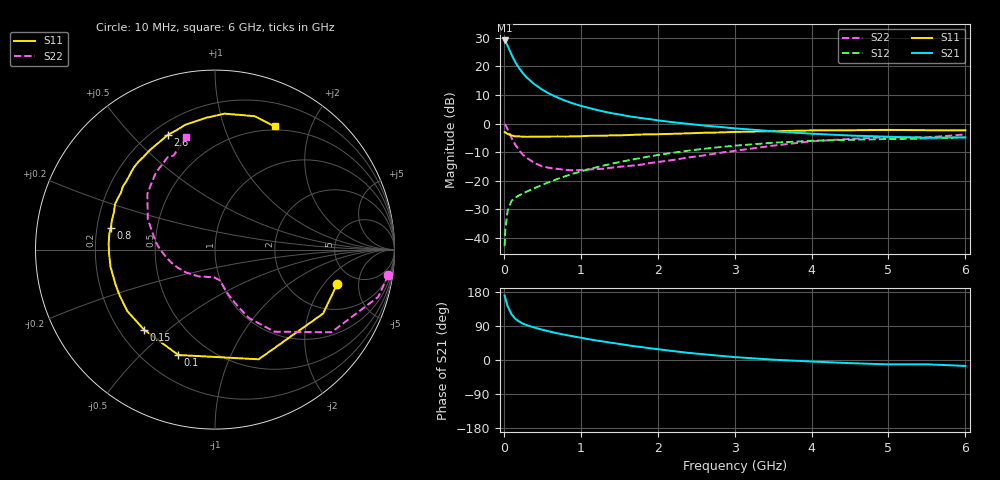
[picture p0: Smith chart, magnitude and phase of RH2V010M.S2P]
! SIEMENS Small Signal Semiconductors
! BFR106
! Si NPN RF Bipolar Junction Transistor in SOT23
! VCE = 2 V  IC = 10 mA
! Common Emitter S-Parameters:  August  1996
# GHz  S  MA  R  50
!  f  S11  S21  S12  S22
! GHz  MAG  ANG  MAG  ANG  MAG  ANG  MAG  ANG
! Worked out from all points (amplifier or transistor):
!   36 points, 10 MHz to 6 GHz, reference 50 ohm
!   highest |S21| = 29.1 dB at 10 MHz (marker M1)
!   |S21| within 3 dB of that: start of sweep to 68.03 MHz
!   unconditionally stable (mu >= 1): 470.6 MHz to 2.33 GHz; 4.596 GHz to end of sweep
!   at 250 MHz: K = 0.72, MSG = 20.9 dB, |S12| = -24.4 dB
!   at 1.4 GHz: K = 1.11, MAG = 6.9 dB, |S12| = -14.0 dB
!   at 6 GHz: K = 1.02, MAG = -0.9 dB, |S12| = -4.8 dB
!   S11 on the Smith chart (normalised r, x): 10 MHz: 3.65, -2.76; 100 MHz: 0.34, -0.65; 150 MHz: 0.30, -0.42; 800 MHz: 0.26, +0.10; 2.6 GHz: 0.26, +0.64; 6 GHz: 0.46, +1.50
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0.01  0.7076 -15.5  28.37 170.4  0.0072 84.3  0.9765 -8.2
0.02  0.6998 -30.6  27.42 162.6  0.0144 77.0  0.9476 -16.1
0.05  0.6577 -68.3  22.78 141.4  0.0304 61.2  0.7955 -35.4
0.1  0.6219 -109.2  16.06 120.6  0.0447 48.5  0.5645 -54.1
0.15  0.596 -131.6  11.76 108.5  0.051 43.6  0.4248 -63.7
0.2  0.5967 -144.8  9.259 101.3  0.0558 44.0  0.3404 -68.1
0.25  0.5898 -153.9  7.513 95.7  0.0606 44.6  0.2825 -71.8
0.3  0.5875 -160.7  6.333 91.8  0.0649 46.6  0.2502 -74.3
0.4  0.5901 -170.6  4.842 85.4  0.0747 50.3  0.2037 -77.8
0.5  0.5905 -177.7  3.903 79.9  0.0849 52.8  0.1787 -80.5
0.6  0.5934 176.7  3.287 74.9  0.0964 55.0  0.1676 -83.4
0.7  0.5954 171.5  2.846 70.3  0.108 56.5  0.1612 -87.5
0.8  0.5936 168.1  2.506 66.3  0.1205 57.3  0.1553 -91.3
1.1  0.6117 155.6  1.883 55.1  0.1583 58.5  0.1578 -104.0
1.3  0.6126 149.1  1.621 48.5  0.1852 57.9  0.1627 -112.8
1.6  0.629 139.7  1.359 39.3  0.2257 55.8  0.1809 -126.8
2.2  0.663 123.1  1.055 23.6  0.3092 48.8  0.231 -154.3
2.6  0.6912 112.3  0.924 15.0  0.3623 42.9  0.2776 -172.0
3.5  0.736 93.9  0.733 0.9  0.463 28.0  0.4117 155.5
4.5  0.7638 79.1  0.618 -8.3  0.5214 11.8  0.5404 127.7
5.5  0.7653 67.9  0.566 -11.4  0.5475 1.7  0.5725 113.8
6  0.7621 64.2  0.574 -15.6  0.5734 -5.4  0.6461 104.5
